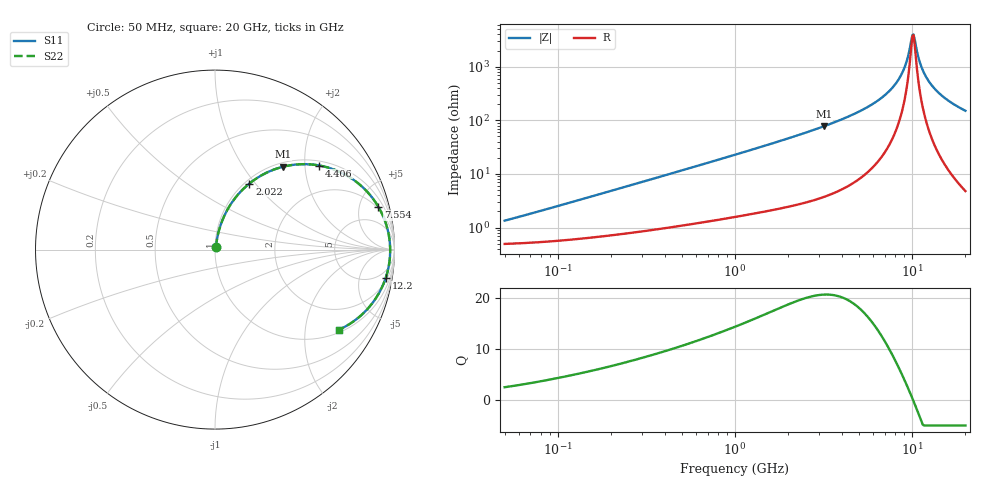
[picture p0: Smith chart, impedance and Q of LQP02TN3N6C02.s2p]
!Murata Part Number: LQP02TN3N6C02
!These Parameters are Measured in Series Mode Connection
!  o--[Z]--o
!Port1  Port2
!  o-------o
!Freq. Start=50[MHz] Stop=20[GHz], 401[Steps]
# Hz S RI R 50
!Freq.(Hz) S11(Real) S11(Imag) S21(Real) S21(Imag) S12(Real) S12(Imag) S22(Real) S22(Imag)
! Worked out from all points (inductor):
!   401 points, 50 MHz to 20 GHz, reference 50 ohm
!   read as one part in series: L = 3.95 nH near 61.67 MHz
!   highest Q = 20.7 at 3.169 GHz (marker M1), where L = 3.87 nH
!   self-resonance near 10.04 GHz
!   S11 on the Smith chart (normalised r, x): 50 MHz: 1.01, +0.03; 2.022 GHz: 1.05, +0.93; 4.406 GHz: 1.12, +2.38; 7.554 GHz: 1.77, +7.37; 12.2 GHz: 3, -12; 20 GHz: 1.10, -3.01
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5e7  0.0051 0.0124  0.9949 -0.0124  0.9949 -0.0124  0.0051 0.0124
1.364002e8  0.00729 0.0328  0.9927 -0.0328  0.9927 -0.0328  0.00729 0.0328
3.721004e8  0.0166 0.0848  0.9834 -0.0848  0.9834 -0.0848  0.0166 0.0848
1e9  0.0626 0.2101  0.9374 -0.2101  0.9374 -0.2101  0.0626 0.2101
2.021818e9  0.1913 0.3677  0.8087 -0.3677  0.8087 -0.3677  0.1913 0.3677
2.728004e9  0.3045 0.4364  0.6955 -0.4364  0.6955 -0.4364  0.3045 0.4364
3.168813e9  0.3792 0.4617  0.6208 -0.4617  0.6208 -0.4617  0.3792 0.4617
4.405649e9  0.5822 0.4683  0.4178 -0.4683  0.4178 -0.4683  0.5822 0.4683
5.944466e9  0.7822 0.3814  0.2178 -0.3814  0.2178 -0.3814  0.7822 0.3814
7.442007e9  0.9042 0.2485  0.0958 -0.2485  0.0958 -0.2485  0.9042 0.2485
7.554318e9  0.9106 0.2378  0.0894 -0.2378  0.0894 -0.2378  0.9106 0.2378
8.264682e9  0.9434 0.1699  0.0566 -0.1699  0.0566 -0.1699  0.9434 0.1699
8.907419e9  0.9624 0.1092  0.0376 -0.1092  0.0376 -0.1092  0.9624 0.1092
9.316812e9  0.97 0.0715  0.03 -0.0715  0.03 -0.0715  0.97 0.0715
9.892087e9  0.9754 0.0204  0.0246 -0.0204  0.0246 -0.0204  0.9754 0.0204
1.004137e10  0.9759 0.00749  0.0241 -0.00749  0.0241 -0.00749  0.9759 0.00749
1.034674e10  0.9759 -0.0183  0.0241 0.0183  0.0241 0.0183  0.9759 -0.0183
1.115139e10  0.9698 -0.0824  0.0302 0.0824  0.0302 0.0824  0.9698 -0.0824
1.220001e10  0.9514 -0.1571  0.0486 0.1571  0.0486 0.1571  0.9514 -0.1571
1.334722e10  0.9217 -0.2275  0.0783 0.2275  0.0783 0.2275  0.9217 -0.2275
1.482269e10  0.8745 -0.3014  0.1255 0.3014  0.1255 0.3014  0.8745 -0.3014
2e10  0.6887 -0.4473  0.3113 0.4473  0.3113 0.4473  0.6887 -0.4473
